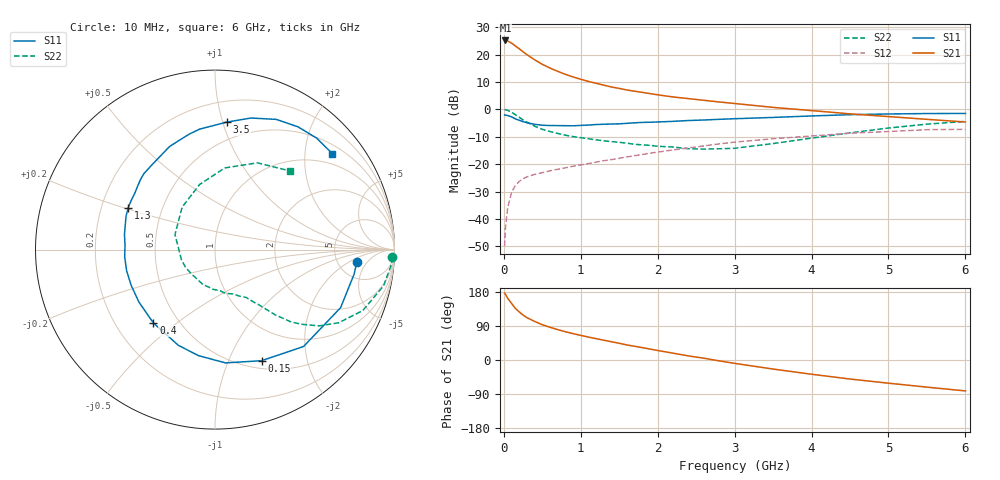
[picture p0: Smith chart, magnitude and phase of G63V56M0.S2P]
! SIEMENS Small Signal Semiconductors
! BFG193
! Si NPN RF Bipolar Junction Transistor in SOT223
! VCE = 3.5 V  IC = 6 mA
! Common Emitter S-Parameters:  August  1996
# GHz  S  MA  R  50
!  f  S11  S21  S12  S22
! GHz  MAG  ANG  MAG  ANG  MAG  ANG  MAG  ANG
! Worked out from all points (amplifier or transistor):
!   36 points, 10 MHz to 6 GHz, reference 50 ohm
!   highest |S21| = 25.2 dB at 20 MHz (marker M1)
!   |S21| within 3 dB of that: start of sweep to 198.3 MHz
!   unconditionally stable (mu >= 1): 1.036 GHz to 2.542 GHz
!   at 250 MHz: K = 0.39, MSG = 23.2 dB, |S12| = -25.3 dB
!   at 1.4 GHz: K = 1.08, MAG = 11.5 dB, |S12| = -18.3 dB
!   at 6 GHz: K = 0.88, MSG = 1.3 dB, |S12| = -7.3 dB
!   S11 on the Smith chart (normalised r, x): 10 MHz: 7.60, -2.84; 150 MHz: 0.59, -1.33; 400 MHz: 0.36, -0.41; 1.3 GHz: 0.32, +0.20; 3.5 GHz: 0.36, +1.03; 6 GHz: 0.71, +2.64
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0.01  0.7934 -5.0  18.1 176.4  0.0032 86.6  0.989 -2.4
0.02  0.7869 -10.1  18.11 173.9  0.0067 85.4  0.9861 -4.9
0.05  0.771 -24.8  17.65 162.8  0.0162 78.5  0.9608 -12.1
0.1  0.7313 -47.6  16.26 149.6  0.0304 68.2  0.8908 -22.4
0.15  0.6713 -67.2  14.36 136.1  0.0411 58.9  0.8007 -30.6
0.2  0.634 -84.7  12.77 126.8  0.0484 53.7  0.7196 -36.2
0.25  0.598 -98.8  11.24 118.5  0.0542 49.0  0.6414 -40.5
0.3  0.5712 -110.9  9.974 111.9  0.0589 46.7  0.5868 -43.5
0.4  0.5338 -130.0  8.058 101.8  0.0652 43.3  0.4941 -47.3
0.5  0.5149 -145.4  6.642 93.1  0.0701 41.7  0.4331 -49.6
0.6  0.5078 -156.8  5.685 86.3  0.0759 41.2  0.395 -51.4
0.7  0.5063 -166.6  4.957 80.2  0.0809 41.5  0.3645 -53.5
0.9  0.5018 177.3  3.912 69.6  0.0919 41.6  0.3193 -56.8
1.1  0.5182 164.8  3.241 60.5  0.1029 42.1  0.2916 -62.5
1.3  0.5367 154.5  2.766 52.2  0.116 41.9  0.2669 -67.8
1.6  0.5577 140.6  2.259 39.7  0.1359 39.9  0.242 -79.4
2.2  0.6056 119.6  1.687 18.0  0.1825 33.5  0.206 -109.0
2.8  0.6598 102.4  1.367 -2.3  0.2351 23.4  0.1916 -149.6
3.5  0.7139 84.6  1.089 -23.9  0.292 8.4  0.2381 159.4
4.5  0.8018 64.8  0.83 -50.2  0.3681 -12.1  0.3728 103.3
5.5  0.8406 47.6  0.659 -71.6  0.4269 -37.4  0.5383 63.9
6  0.8445 39.2  0.589 -81.6  0.4333 -51.9  0.6042 46.6
